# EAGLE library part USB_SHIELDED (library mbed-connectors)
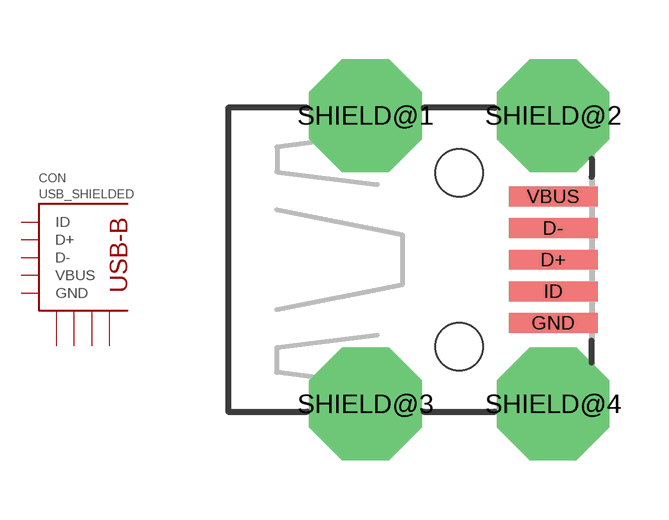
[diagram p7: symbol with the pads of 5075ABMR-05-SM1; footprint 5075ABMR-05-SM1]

Designator prefix CON

## USB_SHIELDED  [5075ABMR-05-SM1]
D+  D+
D-  D-
GND  GND
ID  ID
SHIELD@1  P$1
SHIELD@2  P$2
SHIELD@3  P$3
SHIELD@4  P$4
VBUS  VBUS

## Footprint 5075ABMR-05-SM1 (pad centres in mm)
Neltron 5075ABMR-05-SM1 Mini-USB 5-pin Female Connector
smd 2.25 x 0.5: D+ 2.375,0; D- 2.375,0.8; GND 2.375,-1.6; ID 2.375,-0.8; VBUS 2.375,1.6
drill 1.9 pad 2.5 octagon: SHIELD@1 -2.375,3.65; SHIELD@2 2.375,3.65; SHIELD@3 -2.375,-3.65; SHIELD@4 2.375,-3.65
hole 1.2 at 0,2.2
hole 1.2 at 0,-2.2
